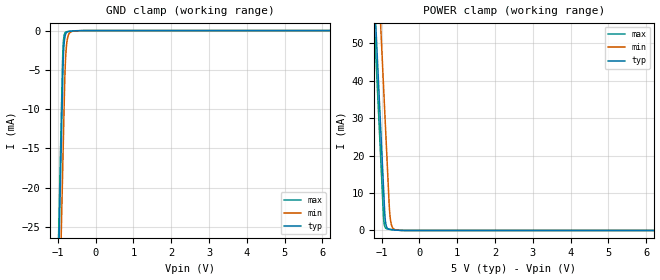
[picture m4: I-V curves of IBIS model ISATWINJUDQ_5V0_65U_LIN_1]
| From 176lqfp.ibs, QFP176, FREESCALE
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[Model] ISATWINJUDQ_5V0_65U_LIN_1
Model_type Input
Polarity   Non-Inverting
| var   typ   min   max
C_comp   1.33815pF  1.32665pF  1.35270pF
Vinl = 800.0mV
Vinh = 2.0V
[Model Spec]
Vinl 800.00000mV 800.00000mV 800.00000mV
Vinh 2.00000V 2.00000V 2.00000V
| variable   typ   min   max
[Temperature Range] 25.0 150.0 -40.0
| variable   typ   min   max
[Voltage Range] 5.0V 4.0V 5.5V
| variable   typ   min   max
[POWER Clamp Reference] 5.0V 4.0V 5.5V
| variable   typ   min   max
[GND Clamp Reference] 0V 0V 0V
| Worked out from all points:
|   GND clamp passes 1 mA (typ) near -0.82 V on its own axis
|   POWER clamp passes 1 mA (typ) near -0.87 V on its own axis
[POWER Clamp]
-5V       872.3mA    899.5mA    864.4mA
-1.24V    73.28mA    100.5mA    65.37mA
-1.16V    56.28mA    83.53mA    48.37mA
-1.09V    41.4mA     68.65mA    33.5mA
-1.01V    24.4mA     51.65mA    16.5mA
-940mV    9.527mA    36.78mA    2.492mA
-910mV    3.699mA    30.4mA     925.2uA
-860mV    810.5uA    19.78mA    449.2uA
-800mV    309.8uA    7.027mA    334.4uA
-770mV    244.7uA    3.216mA    294.8uA
-610mV    88.57uA    136.9uA    114.5uA
10V       0A         0A         0A
[GND Clamp]
-5V       -883.8mA   -895.1mA   -880.4mA
-1.01V    -35.94mA   -47.19mA   -32.5mA
-880mV    -8.313mA   -19.57mA   -4.877mA
-860mV    -4.257mA   -15.32mA   -1.922mA
-840mV    -2.053mA   -11.07mA   -815.4uA
-810mV    -747.2uA   -5.25mA    -294.1uA
-790mV    -418.9uA   -3.108mA   -190.1uA
-770mV    -261.3uA   -1.862mA   -146.7uA
-730mV    -141.8uA   -708.2uA   -115.2uA
-670mV    -88.94uA   -211.7uA   -87.52uA
-310mV    -77.67nA   -778.4nA   -24.16nA
10V       417.1pA    58.73nA    262.7pA
